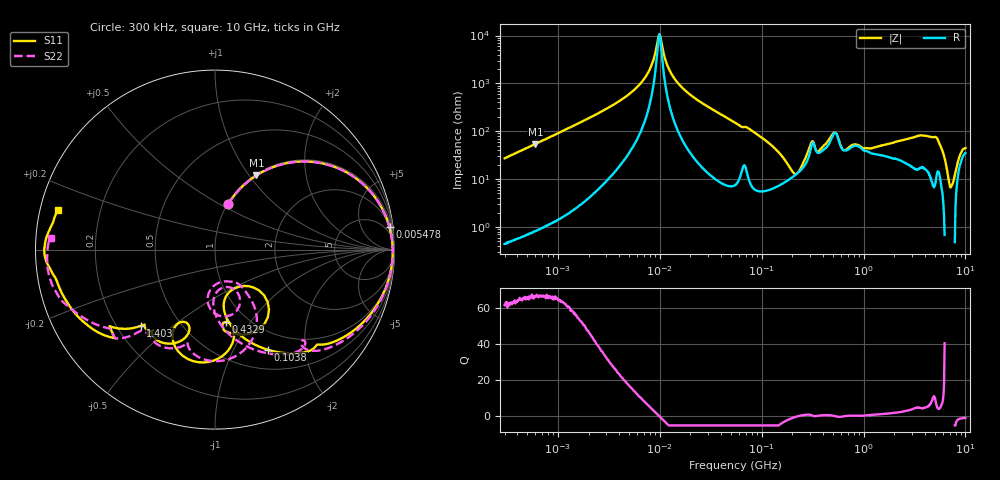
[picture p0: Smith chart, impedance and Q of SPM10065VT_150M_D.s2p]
! S-Parameter Data Generated by TDK Corporation
! Copyright(C) 2020 TDK Corporation.
! All Rights Reserved.
! TDK P/N: SPM10065VT-150M-D (Inductor)
! Property: L=15uH at 100kHz
! Size(LxWxT): 10.5x10x6.5mm
! Model Type: s2p (Touchstone File Format Version 1.0)
! Frequency: DC=Yes Start=0.3MHz Stop=10000MHz 802points Log-sweep
! Model Generated on Apr. 23, 2020
! Port Assignments:
!  1 ---@@@--- 2
! Applicable Conditions:
!  Temperature = 25 degC
!  DC Bias Current = 0 A
!  Small Signal Operation
! Terms and conditions regarding TDK Simulation Models
! (1)This simulation model is being provided solely for informational purposes. Please refer to the specifications of the products in terms of detailed characteristics of such products.
! (2)In no event shall TDK Corporation of any of its subsidiaries be liable for any loss or damage arising, directly or indirectly,
!  From any information contained in this simulation model, including, but not limited to loss or damages arising from any inaccuracies, omissions or errors in connection with such information.
! (3)Any and all copyrights on this simulation model are owned by TDK Corporation.
!  Duplication or redistribution of this simulation model without prior written permission from TDK Corporation is prohibited.
! (4)This simulation model is subject to any modification or change without any prior notice.
! (5)Neither TDK Corporation nor any of its subsidiaries shall make any warranty, express or implied,
!  Including but not limited to the correctness, implied warranties of merchantability and fitness for a particular purpose with respect to this simulation models.
! (6)The use of this simulation model shall be deemed to have consented to the terms and conditions hereof.
# Hz S MA R 50
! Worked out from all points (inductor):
!   801 points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, 300 kHz to 10 GHz, reference 50 ohm
!   read as one part in series: L = 14.3 uH near 318.3 kHz
!   highest Q = 66.7 at 601.5 kHz (marker M1), where L = 14.4 uH
!   self-resonance near 9.909 MHz
!   S11 on the Smith chart (normalised r, x): 300 kHz: 1.01, +0.54; 5.478 MHz: 2, +15; 103.8 MHz: 0.74, -1.38; 432.9 MHz: 0.80, -0.77; 1.403 GHz: 0.30, -0.39; 10 GHz: 0.05, +0.12
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300000  0.2618 74.1  0.9606 -15.1  0.9608 -15.1  0.2617 74.0
601544  0.4737 60.8  0.8738 -28.3  0.8737 -28.3  0.4737 60.8
1713600  0.8372 31.8  0.531 -57.1  0.5308 -57.1  0.8374 31.7
5478281  0.9803 7.3  0.1401 -78.9  0.14 -78.9  0.9806 7.0
8009306  0.9892 1.7  0.04935 -77.4  0.04938 -77.5  0.9894 1.3
9671944  0.9904 -1.0  0.01103 -32.9  0.01104 -33.0  0.9905 -1.5
1.257005e7  0.9888 -4.8  0.05429 74.9  0.05428 74.9  0.9889 -5.4
1.626666e7  0.9834 -8.8  0.1152 75.9  0.1152 75.9  0.9835 -9.7
5.477226e7  0.8342 -38.3  0.5178 47.1  0.5176 47.1  0.8251 -42.3
1.038383e8  0.6321 -62.1  0.7351 22.5  0.7348 22.5  0.6269 -65.5
1.990845e8  0.3554 -81.3  0.8426 -12.3  0.8422 -12.3  0.3338 -91.0
2.756623e8  0.2424 -64.4  0.778 -37.0  0.7777 -37.0  0.2182 -72.8
3.126428e8  0.4122 -44.8  0.5738 -44.7  0.5736 -44.7  0.3639 -71.0
3.7738e8  0.4708 -80.1  0.6308 -45.0  0.6306 -45.0  0.1848 -81.8
4.329008e8  0.4081 -81.6  0.5731 -53.3  0.5728 -53.3  0.2796 -53.9
5.105874e8  0.5979 -86.6  0.4102 -60.8  0.41 -60.8  0.4874 -61.7
5.911415e8  0.5674 -114.1  0.4458 -46.0  0.4456 -46.0  0.6215 -87.6
7.318083e8  0.4679 -107.7  0.4915 -67.6  0.4913 -67.6  0.5382 -106.5
1.403063e9  0.592 -134.2  0.3319 -119.1  0.3317 -119.1  0.6126 -132.3
1.767019e9  0.6762 -139.3  0.2351 -146.8  0.235 -146.8  0.6892 -135.1
5.157474e9  0.9021 -169.8  0.01663 158.3  0.01657 158.0  0.9189 -165.6
1e10  0.9039 166.0  0.01568 135.4  0.0156 135.7  0.9141 175.8
